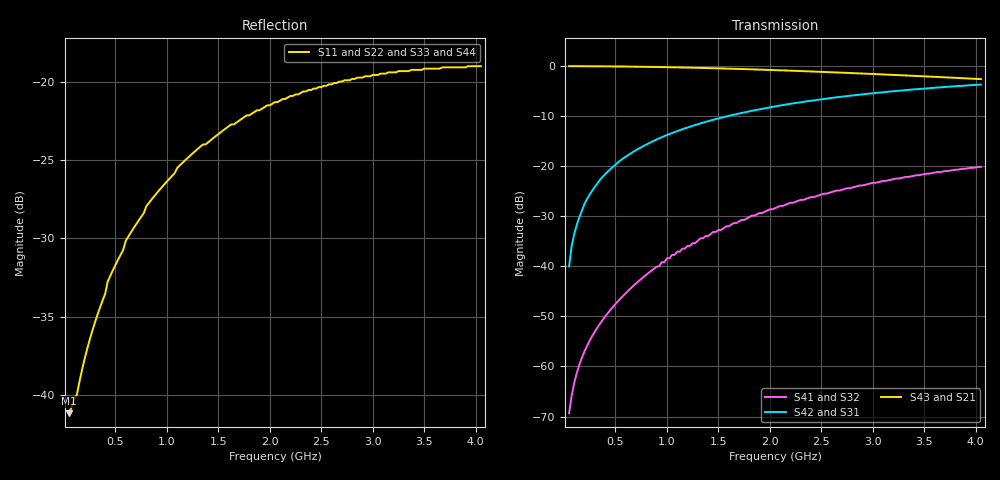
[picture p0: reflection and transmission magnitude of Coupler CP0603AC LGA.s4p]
!	AVX THIN FILM OPERATION
!	CP0603 HIGH DIRECTIVITY COUPLERS
!	P/N CP0603AxxxxCLTR
!	Network	Analyzer HP8720ES.07.64:Feb23,2000 Serial No.US39172382
!	Hewlett-Packard
!	24 July 2003	02:45:57
# MHZ S MA R 50
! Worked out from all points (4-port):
!   161 points, 50 MHz to 4.05 GHz, reference 50 ohm
!   strongest paths, dB at 50 MHz, 1.05 GHz, 2.05 GHz, 3.05 GHz, 4.05 GHz:
!     S43: -0.1, -0.3, -0.9, -1.7, -2.7
!     S21: -0.1, -0.3, -0.9, -1.7, -2.7
!     S42: -40.0, -13.4, -8.1, -5.4, -3.7
!     S31: -40.0, -13.4, -8.1, -5.4, -3.7
!     S41: -69.3, -37.7, -28.4, -23.2, -20.2
!     S32: -69.3, -37.7, -28.4, -23.2, -20.2
!   lowest |S11| = -41.2 dB at 50 MHz (marker M1), VSWR 1.02, Z = 50.8 - j0.261 ohm
!   |S11| at or under -10 dB: start of sweep to end of sweep
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50  0.008732 -17.1  0.992 -0.5  0.01 89.5  0.0003411 84.8
    0.992 -0.5  0.008732 -17.1  0.0003411 84.8  0.01 89.5
    0.01 89.5  0.0003411 84.8  0.008732 -17.1  0.992 -0.5
    0.0003411 84.8  0.01 89.5  0.992 -0.5  0.008732 -17.1
75  0.009164 -24.9  0.991 -0.7  0.016 89.3  0.0005134 82.4
    0.991 -0.7  0.009164 -24.9  0.0005134 82.4  0.016 89.3
    0.016 89.3  0.0005134 82.4  0.009164 -24.9  0.991 -0.7
    0.0005134 82.4  0.016 89.3  0.991 -0.7  0.009164 -24.9
150  0.011 -43.4  0.991 -1.4  0.031 88.6  0.001045 75.2
     0.991 -1.4  0.011 -43.4  0.001045 75.2  0.031 88.6
     0.031 88.6  0.001045 75.2  0.011 -43.4  0.991 -1.4
     0.001045 75.2  0.031 88.6  0.991 -1.4  0.011 -43.4
350  0.019 -68.1  0.989 -3.3  0.073 86.7  0.002673 57.8
     0.989 -3.3  0.019 -68.1  0.002673 57.8  0.073 86.7
     0.073 86.7  0.002673 57.8  0.019 -68.1  0.989 -3.3
     0.002673 57.8  0.073 86.7  0.989 -3.3  0.019 -68.1
1100  0.053 -92.7  0.965 -10.2  0.223 79.7  0.014 17.4
      0.965 -10.2  0.053 -92.7  0.014 17.4  0.223 79.7
      0.223 79.7  0.014 17.4  0.053 -92.7  0.965 -10.2
      0.014 17.4  0.223 79.7  0.965 -10.2  0.053 -92.7
2300  0.092 -107.5  0.887 -20.4  0.433 69.5  0.046 -11.3
      0.887 -20.4  0.092 -107.5  0.046 -11.3  0.433 69.5
      0.433 69.5  0.046 -11.3  0.092 -107.5  0.887 -20.4
      0.046 -11.3  0.433 69.5  0.887 -20.4  0.092 -107.5
4050  0.112 -117.8  0.737 -32.5  0.65 57.6  0.098 -33.1
      0.737 -32.5  0.112 -117.8  0.098 -33.1  0.65 57.6
      0.65 57.6  0.098 -33.1  0.112 -117.8  0.737 -32.5
      0.098 -33.1  0.65 57.6  0.737 -32.5  0.112 -117.8
